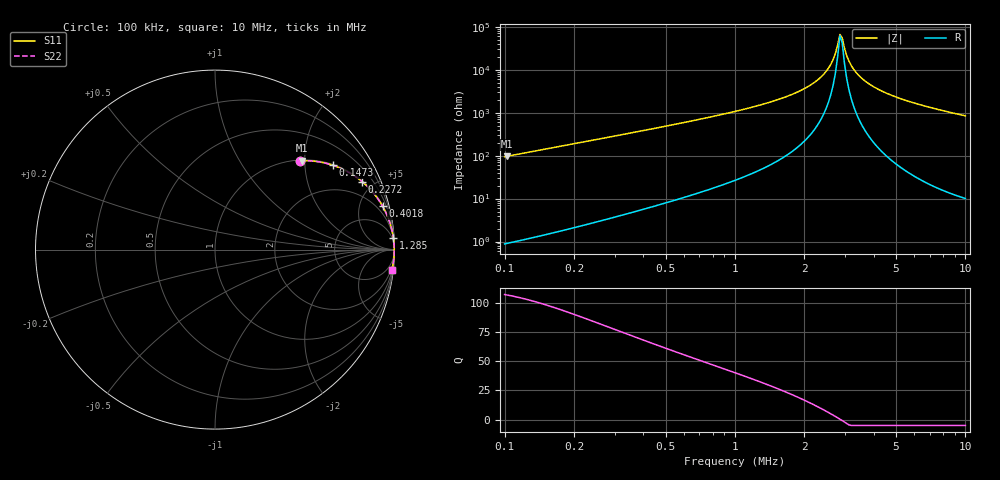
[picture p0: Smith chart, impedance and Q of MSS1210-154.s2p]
# MHz S MA R 50
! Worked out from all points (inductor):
!   203 points, 100 kHz to 10 MHz, reference 50 ohm
!   read as one part in series: L = 150 uH near 102.3 kHz
!   highest Q = 107 at 102.3 kHz (marker M1), where L = 150 uH
!   self-resonance near 2.854 MHz
!   S11 on the Smith chart (normalised r, x): 100 kHz: 1.02, +1.89; 147.3 kHz: 1.03, +2.78; 227.2 kHz: 1.05, +4.31; 401.8 kHz: 1.11, +7.71; 1.285 MHz: 2, +30; 10 MHz: 1, -17
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0.1  0.6831 46.4  0.724 -43.1  0.724 -43.1  0.6831 46.4
0.102306  0.6913 45.7  0.7161 -43.7  0.7161 -43.7  0.6913 45.7
0.1473387  0.8082 35.5  0.5807 -53.9  0.5807 -53.9  0.8082 35.5
0.2272143  0.903 24.8  0.4194 -64.5  0.4194 -64.5  0.903 24.8
0.4017542  0.9645 14.5  0.2501 -74.7  0.2501 -74.7  0.9645 14.5
0.7435105  0.9886 7.6  0.1319 -81.3  0.1319 -81.3  0.9886 7.6
1.285023  0.9958 3.8  0.06598 -84.5  0.06598 -84.5  0.9958 3.8
1.768173  0.9976 2.1  0.03735 -85.2  0.03735 -85.2  0.9976 2.1
2.220929  0.9982 1.1  0.01935 -84.3  0.01935 -84.3  0.9982 1.1
2.546482  0.9985 0.5  0.009108 -80.2  0.009108 -80.2  0.9985 0.5
2.726739  0.9986 0.2  0.004167 -69.7  0.004167 -69.7  0.9986 0.2
2.853945  0.9986 0.0  0.001504 -21.1  0.001504 -21.1  0.9986 0.0
2.919756  0.9986 -0.1  0.001801 39.4  0.001801 39.4  0.9986 -0.1
2.987085  0.9986 -0.2  0.003148 63.9  0.003148 63.9  0.9986 -0.2
3.126436  0.9986 -0.4  0.006353 77.3  0.006353 77.3  0.9986 -0.4
3.424944  0.9986 -0.7  0.01307 83.5  0.01307 83.5  0.9986 -0.7
3.751953  0.9985 -1.1  0.01996 85.2  0.01996 85.2  0.9985 -1.1
4.110185  0.9984 -1.5  0.02702 85.8  0.02702 85.8  0.9984 -1.5
5.162633  0.9978 -2.6  0.04578 85.9  0.04578 85.9  0.9978 -2.6
6.787083  0.9963 -4.1  0.07146 85.0  0.07146 85.0  0.9963 -4.1
8.524974  0.994 -5.6  0.09673 83.7  0.09673 83.7  0.994 -5.6
10  0.9917 -6.7  0.1172 82.6  0.1172 82.6  0.9917 -6.7
